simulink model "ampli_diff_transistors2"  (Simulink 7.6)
settings: Solver=ode15s  StartTime=0.0  StopTime=.04  RelTol=1e-3
StopFcn:
  | close all, clc
  | load  ES_ampli_diff.mat
  | plotyy(x(1,:),x(2,:),x(1,:),x(3,:))
  | grid
  | title('Tension de sortie et courant de collecteur - Ampli différentiel')
  | xlabel('temps')
libraries: fl_lib x16, elec_lib x5, nesl_utility x4

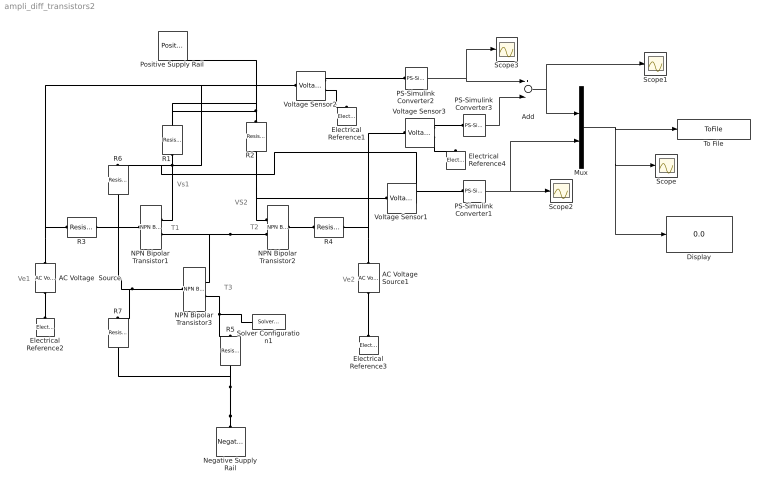
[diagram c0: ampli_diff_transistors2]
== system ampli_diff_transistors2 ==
  note: T1
  note: T2
  note: T3
  note: Vs1
  note: VS2
  note: Ve1
  note: Ve2
  AC Voltage  Source : fl_lib/Electrical/Electrical Sources/AC Voltage Source  DialogController=NetworkEngine.DynNeDlgSource  SystemSampleTime=-1  amp=0.1 V  shift=0 rad  omega=60 Hz  i_Log=off  v_Log=off  LocalVarNames=|current|voltage|power  LocalVarDescs=|Current (A)|Voltage (V)|Power (W)  LocalVarLogging=[0 0 0]
  AC Voltage  Source1 : fl_lib/Electrical/Electrical Sources/AC Voltage Source  DialogController=NetworkEngine.DynNeDlgSource  SystemSampleTime=-1  amp=.11 V  shift=0 rad  omega=60 Hz  i_Log=off  v_Log=off  LocalVarNames=|current|voltage|power  LocalVarDescs=|Current (A)|Voltage (V)|Power (W)  LocalVarLogging=[0 0 0]
  Add : Sum  Inputs=+-
  Display : Display
  Electrical Reference{1..4} (4 alike) : fl_lib/Electrical/Electrical Elements/Electrical Reference  DialogController=NetworkEngine.DynNeDlgSource  SystemSampleTime=-1  i_Log=off  LocalVarNames=|i  LocalVarDescs=|i  LocalVarLogging=[]
  Mux : Mux  Inputs=2
  NPN Bipolar Transistor1 : elec_lib/Semiconductor Devices/NPN Bipolar Transistor  DialogController=NetworkEngine.DynNeDlgSource  SystemSampleTime=-1  parameterization=1  BF=100  IS=1e-14 A  VAF=200 V  hfe=100  hoe=5e-5 1/Ohm  Ic_h=1 mA  V1=0.55 V  I1=0.5 mA  BR=1  Tmeas=25 C  RC=0.01 Ohm  RE=1e-4 Ohm  RB=1 Ohm  C_BC=5 pF  C_BE=5 pF  TF=0 us  TR=0 us  LocalVarLogging=[]
  NPN Bipolar Transistor2 : elec_lib/Semiconductor Devices/NPN Bipolar Transistor  DialogController=NetworkEngine.DynNeDlgSource  SystemSampleTime=-1  parameterization=1  BF=100  IS=1e-14 A  VAF=200 V  hfe=100  hoe=5e-5 1/Ohm  Ic_h=1 mA  V1=0.55 V  I1=0.5 mA  BR=1  Tmeas=25 C  RC=0.01 Ohm  RE=1e-4 Ohm  RB=1 Ohm  C_BC=5 pF  C_BE=5 pF  TF=0 us  TR=0 us  LocalVarLogging=[]
  NPN Bipolar Transistor3 : elec_lib/Semiconductor Devices/NPN Bipolar Transistor  DialogController=NetworkEngine.DynNeDlgSource  SystemSampleTime=-1  parameterization=1  BF=100  IS=1e-14 A  VAF=200 V  hfe=100  hoe=5e-5 1/Ohm  Ic_h=1 mA  V1=0.55 V  I1=0.5 mA  BR=1  Tmeas=25 C  RC=0.01 Ohm  RE=1e-4 Ohm  RB=1 Ohm  C_BC=5 pF  C_BE=5 pF  TF=0 us  TR=0 us  LocalVarLogging=[]
  Negative Supply Rail : elec_lib/Sources/Negative Supply Rail  DialogController=NetworkEngine.DynNeDlgSource  SystemSampleTime=-1  v0=-24 V  current_Log=off  voltage_Log=off  power_Log=off  LocalVarNames=|current|voltage|power  LocalVarDescs=|Current (A)|Voltage (V)|Power (W)  LocalVarLogging=[0 0 0]
  PS-Simulink Converter1 : nesl_utility/PS-Simulink Converter  DialogController=NetworkEngine.DynNeUtilDlgSource  SystemSampleTime=-1  PhysicalDomain=network_engine_domain  LeftPortType=input  RightPortType=output  SubClassName=ps_output  Unit=1  AffineConversion=off
  PS-Simulink Converter2 : nesl_utility/PS-Simulink Converter  DialogController=NetworkEngine.DynNeUtilDlgSource  SystemSampleTime=-1  PhysicalDomain=network_engine_domain  LeftPortType=input  RightPortType=output  SubClassName=ps_output  Unit=1  AffineConversion=off
  PS-Simulink Converter3 : nesl_utility/PS-Simulink Converter  DialogController=NetworkEngine.DynNeUtilDlgSource  SystemSampleTime=-1  PhysicalDomain=network_engine_domain  LeftPortType=input  RightPortType=output  SubClassName=ps_output  Unit=1  AffineConversion=off
  Positive Supply Rail : elec_lib/Sources/Positive Supply Rail  DialogController=NetworkEngine.DynNeDlgSource  SystemSampleTime=-1  v0=24 V  current_Log=off  voltage_Log=off  power_Log=off  LocalVarNames=|current|voltage|power  LocalVarDescs=|Current (A)|Voltage (V)|Power (W)  LocalVarLogging=[0 0 0]
  R1 : fl_lib/Electrical/Electrical Elements/Resistor  DialogController=NetworkEngine.DynNeDlgSource  SystemSampleTime=-1  R=4.7 kOhm  i_Log=off  v_Log=off  LocalVarNames=|current|voltage|power  LocalVarDescs=|Resistor current (A)|Voltage across resistor (V)|Power (W)  LocalVarLogging=[0 0 0]
  R2 : fl_lib/Electrical/Electrical Elements/Resistor  DialogController=NetworkEngine.DynNeDlgSource  SystemSampleTime=-1  R=4.7 kOhm  i_Log=off  v_Log=off  LocalVarNames=|current|voltage|power  LocalVarDescs=|Resistor current (A)|Voltage across resistor (V)|Power (W)  LocalVarLogging=[0 0 0]
  R3 : fl_lib/Electrical/Electrical Elements/Resistor  DialogController=NetworkEngine.DynNeDlgSource  SystemSampleTime=-1  R=100 Ohm  i_Log=off  v_Log=off  LocalVarNames=|current|voltage|power  LocalVarDescs=|Resistor current (A)|Voltage across resistor (V)|Power (W)  LocalVarLogging=[0 0 0]
  R4 : fl_lib/Electrical/Electrical Elements/Resistor  DialogController=NetworkEngine.DynNeDlgSource  SystemSampleTime=-1  R=100 Ohm  i_Log=off  v_Log=off  LocalVarNames=|current|voltage|power  LocalVarDescs=|Resistor current (A)|Voltage across resistor (V)|Power (W)  LocalVarLogging=[0 0 0]
  R5 : fl_lib/Electrical/Electrical Elements/Resistor  DialogController=NetworkEngine.DynNeDlgSource  SystemSampleTime=-1  R=22 Ohm  i_Log=off  v_Log=off  LocalVarNames=|current|voltage|power  LocalVarDescs=|Resistor current (A)|Voltage across resistor (V)|Power (W)  LocalVarLogging=[0 0 0]
  R6 : fl_lib/Electrical/Electrical Elements/Resistor  DialogController=NetworkEngine.DynNeDlgSource  SystemSampleTime=-1  R=22 kOhm  i_Log=off  v_Log=off  LocalVarNames=|current|voltage|power  LocalVarDescs=|Resistor current (A)|Voltage across resistor (V)|Power (W)  LocalVarLogging=[0 0 0]
  R7 : fl_lib/Electrical/Electrical Elements/Resistor  DialogController=NetworkEngine.DynNeDlgSource  SystemSampleTime=-1  R=4.7 kOhm  i_Log=off  v_Log=off  LocalVarNames=|current|voltage|power  LocalVarDescs=|Resistor current (A)|Voltage across resistor (V)|Power (W)  LocalVarLogging=[0 0 0]
  Scope{,1..3} (4 alike) : Scope
  Solver Configuration1 : nesl_utility/Solver Configuration  DialogController=NetworkEngine.DynNeUtilDlgSource  SystemSampleTime=-1  PhysicalDomain=network_engine_domain  LeftPortType=input  RightPortType=generic  SubClassName=solver  Accelerate=off  Profile=off  ResidualTolerance=1e-9  MaxNonlinIter=12  MaxModeIter=2  DoFixedCost=off  UseLocalSampling=off  DoDC=off  LinearAlgebra=Sparse  LocalSolverSampleTime=.001  LocalSolverChoice=NE_BACKWARD_EULER_ADVANCER  UseLocalSolver=off
  To File : ToFile  Filename=ES_ampli_diff  MatrixName=x
  Voltage Sensor1 : fl_lib/Electrical/Electrical Sensors/Voltage Sensor  DialogController=NetworkEngine.DynNeDlgSource  SystemSampleTime=-1  i1_Log=off  v1_Log=off  LocalVarNames=|i1|v1  LocalVarDescs=|i1|v1  LocalVarLogging=[]
  Voltage Sensor2 : fl_lib/Electrical/Electrical Sensors/Voltage Sensor  DialogController=NetworkEngine.DynNeDlgSource  SystemSampleTime=-1  i1_Log=off  v1_Log=off  LocalVarNames=|i1|v1  LocalVarDescs=|i1|v1  LocalVarLogging=[]
  Voltage Sensor3 : fl_lib/Electrical/Electrical Sensors/Voltage Sensor  DialogController=NetworkEngine.DynNeDlgSource  SystemSampleTime=-1  i1_Log=off  v1_Log=off  LocalVarNames=|i1|v1  LocalVarDescs=|i1|v1  LocalVarLogging=[]
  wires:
  Mux/1 -> To File/1, Scope/1, Display/1
  PS-Simulink Converter1/1 -> Mux/2, Scope2/1
  PS-Simulink Converter2/1 -> Add/1, Scope3/1
  PS-Simulink Converter3/1 -> Add/2
  Add/1 -> Mux/1, Scope1/1
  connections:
  NPN Bipolar Transistor2/RConn2 -- NPN Bipolar Transistor1/RConn2 -- NPN Bipolar Transistor3/RConn1
  R1/RConn1 -- NPN Bipolar Transistor1/RConn1 -- Voltage Sensor1/RConn2
  R2/RConn1 -- NPN Bipolar Transistor2/RConn1 -- Voltage Sensor1/LConn1
  AC Voltage  Source/LConn1 -- R3/LConn1 -- Voltage Sensor2/LConn1
  R3/RConn1 -- NPN Bipolar Transistor1/LConn1
  AC Voltage  Source/RConn1 -- Electrical Reference2/LConn1
  Electrical Reference3/LConn1 -- AC Voltage  Source1/RConn1
  AC Voltage  Source1/LConn1 -- R4/RConn1 -- Voltage Sensor3/LConn1
  NPN Bipolar Transistor2/LConn1 -- R4/LConn1
  R2/LConn1 -- R1/LConn1 -- Positive Supply Rail/RConn1 -- R6/LConn1
  Voltage Sensor1/RConn1 -- PS-Simulink Converter1/LConn1
  Negative Supply Rail/LConn1 -- R5/RConn1 -- R7/RConn1
  NPN Bipolar Transistor3/LConn1 -- R7/LConn1 -- R6/RConn1
  Voltage Sensor2/RConn1 -- PS-Simulink Converter2/LConn1
  Voltage Sensor2/RConn2 -- Electrical Reference1/LConn1
  NPN Bipolar Transistor3/RConn2 -- R5/LConn1 -- Solver Configuration1/RConn1
  Voltage Sensor3/RConn2 -- Electrical Reference4/LConn1
  Voltage Sensor3/RConn1 -- PS-Simulink Converter3/LConn1
